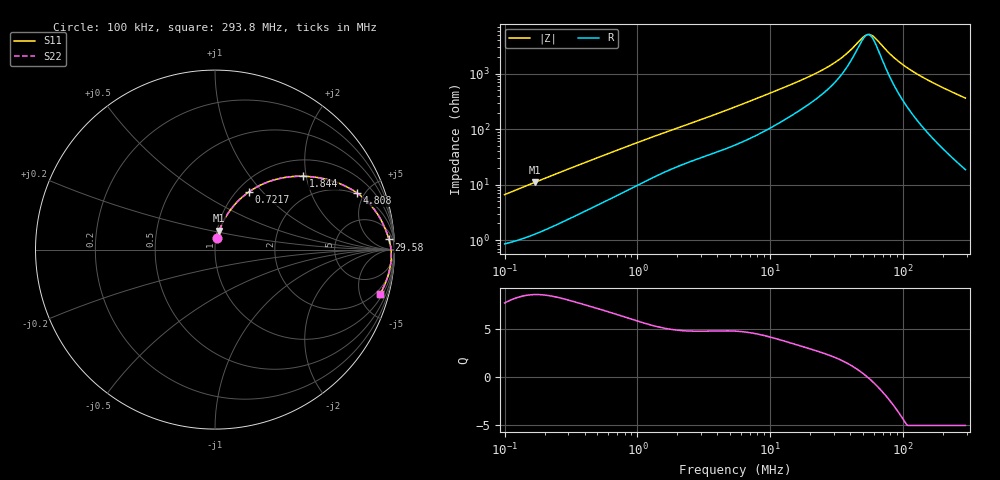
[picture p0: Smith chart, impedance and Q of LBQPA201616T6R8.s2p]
! LBQPA201616T6R8  S-PARAMETER MODEL  ( General Type )
! Model Generated by TAIYO YUDEN Corporation (http://www.ty-top.com)
! Version 1.0
! TAIYO YUDEN Control No. 191025NI43SB-FBB
! Copyright(c) 2019 TAIYO YUDEN CO.,LTD. All Rights Reserved.
! Product Description (link to TY-COMPAS)
! https://ds.yuden.co.jp/TYCOMPAS/or/detail?pn=LBQPA201616T6R8M&u=M
! Products Name : Inductors
! Characteristics :
!  Inductance : 6.8 uH , SRF(min) : 38 MHz , DC Resistance(max) : 0.767 Ohm
!  Rated Current : Saturation :450 mA , Temp Rise : 360 mA (20 degC)
!  Case Size : 2.0 x 1.6 / 0.079 x 0.063 [mm/inch] , Thickness : 1.6 / 0.063 [mm/inch]
!  (Conditions: Temperature = 25 degC , DC Bias Current/Voltage = 0A / 0V)
! External Node Assignments :
!  1  o---GGG---o  2
! GND o---------o GND
! Frequency Range : 0.1MHz  -  293.796821MHz  [ 402 STEP ]
# MHz S RI R 50
! Freq[MHz].  S11 Real  S11 Imag  S21 Real  S21 Imag  S12 Real  S12 Imag  S22 Real  S22 Imag
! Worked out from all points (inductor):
!   401 points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, 100 kHz to 293.8 MHz, reference 50 ohm
!   read as one part in series: L = 10.4 uH near 104.1 kHz
!   highest Q = 8.56 at 168 kHz (marker M1), where L = 10.3 uH
!   self-resonance near 53.99 MHz
!   S11 on the Smith chart (normalised r, x): 100 kHz: 1.02, +0.13; 721.7 kHz: 1.13, +0.85; 1.844 MHz: 1.39, +1.92; 4.808 MHz: 1.92, +4.42; 29.58 MHz: 14, +27; 293.8 MHz: 1.37, -7.28
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0.1  0.0126 0.0641  0.9874 -0.0641  0.9874 -0.0641  0.0126 0.0641
0.168044  0.0238 0.1047  0.9762 -0.1047  0.9762 -0.1047  0.0238 0.1047
0.380976  0.0782 0.2106  0.9218 -0.2106  0.9218 -0.2106  0.0782 0.2106
0.721675  0.1895 0.3219  0.8105 -0.3219  0.8105 -0.3219  0.1895 0.3219
1.451429  0.4066 0.4043  0.5934 -0.4043  0.5934 -0.4043  0.4066 0.4043
1.844324  0.4919 0.4088  0.5081 -0.4088  0.5081 -0.4088  0.4919 0.4088
2.919106  0.6495 0.3836  0.3505 -0.3836  0.3505 -0.3836  0.6495 0.3836
4.808425  0.7921 0.3148  0.2079 -0.3148  0.2079 -0.3148  0.7921 0.3148
5.420303  0.8192 0.2941  0.1808 -0.2941  0.1808 -0.2941  0.8192 0.2941
9.670679  0.9087 0.1928  0.0913 -0.1928  0.0913 -0.1928  0.9087 0.1928
20.65007  0.9574 0.0924  0.0426 -0.0924  0.0426 -0.0924  0.9574 0.0924
29.579  0.9694 0.0564  0.0306 -0.0564  0.0306 -0.0564  0.9694 0.0564
36.84299  0.9748 0.0358  0.0252 -0.0358  0.0252 -0.0358  0.9748 0.0358
49.70575  0.9798 0.00787  0.0202 -0.00787  0.0202 -0.00787  0.9798 0.00787
53.83777  0.9807 0.000271  0.0193 -0.000271  0.0193 -0.000271  0.9807 0.000271
57.16069  0.9813 -0.00551  0.0187 0.00551  0.0187 0.00551  0.9813 -0.00551
60.68869  0.9817 -0.0114  0.0183 0.0114  0.0183 0.0114  0.9817 -0.0114
78.67184  0.9822 -0.038  0.0178 0.038  0.0178 0.038  0.9822 -0.038
99.96794  0.9804 -0.0651  0.0196 0.0651  0.0196 0.0651  0.9804 -0.0651
132.2033  0.975 -0.1015  0.025 0.1015  0.025 0.1015  0.975 -0.1015
197.081  0.9574 -0.1658  0.0426 0.1658  0.0426 0.1658  0.9574 -0.1658
293.7968  0.919 -0.2484  0.081 0.2484  0.081 0.2484  0.919 -0.2484
